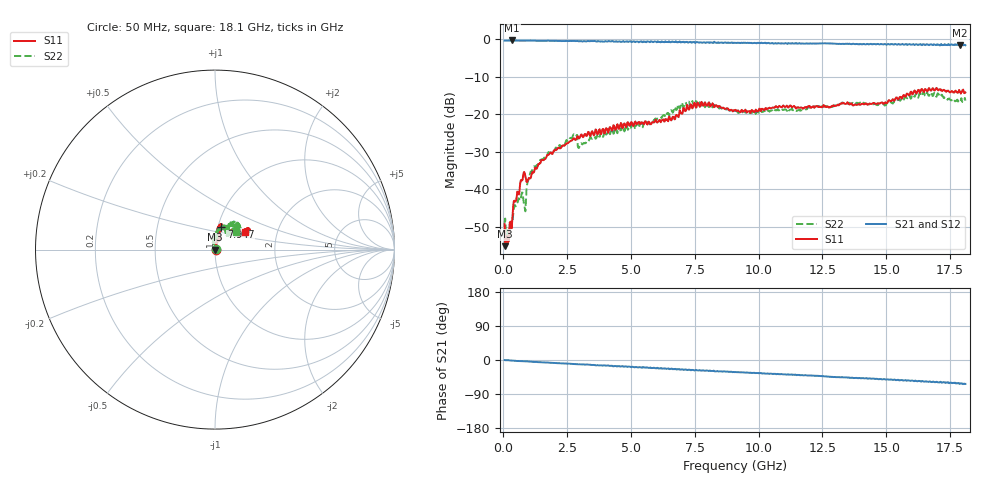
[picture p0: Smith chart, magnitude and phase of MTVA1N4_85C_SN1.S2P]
! Network Analyzer HP8720D.06.14 Serial No. US36140669
! 12 Jan 2005  09:00:05
! Frequency  S11  S21  S12  S22
# HZ  S  DB R 50
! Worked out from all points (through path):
!   801 points, 50 MHz to 18.1 GHz, reference 50 ohm
!   highest |S21| = -0.36 dB at 343.3 MHz (marker M1); lowest = -1.7 dB at 17.9 GHz (marker M2)
!   group delay of S21, straight-line fit = 9.33 ps
!   lowest |S11| = -55.1 dB at 72.56 MHz (marker M3), VSWR 1.00, Z = 50.1 - j0.101 ohm
!   |S11| at or under -10 dB: start of sweep to end of sweep
!   |S22| runs from -53.5 to -14.1 dB; largest |S21 - S12| = 0.032
!   S11 on the Smith chart (normalised r, x): 50 MHz: 1.01, -0.00; 7.947 GHz: 1.04, +0.27; 18.1 GHz: 1.37, +0.28
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5e7  -49.23 -2.3  -0.41 -0.2  -0.39 -0.6  -48.90 34.6
7.25625e7  -55.10 -34.8  -0.43 -0.4  -0.40 -0.7  -47.76 -15.5
1.628125e8  -52.34 58.2  -0.41 -0.5  -0.41 -0.9  -50.81 43.9
3.433125e8  -48.82 71.7  -0.36 -1.5  -0.38 -1.8  -48.94 57.1
5.238125e8  -41.96 87.7  -0.42 -2.6  -0.41 -2.8  -43.70 71.9
7.494375e8  -37.50 80.7  -0.46 -3.2  -0.44 -3.4  -40.84 69.7
8.6225e8  -36.39 60.8  -0.44 -3.5  -0.42 -3.8  -45.83 115.4
1.020188e9  -37.08 70.6  -0.43 -4.0  -0.41 -4.4  -36.63 109.2
1.22325e9  -34.88 84.5  -0.44 -5.2  -0.44 -5.4  -34.00 103.8
1.787312e9  -30.69 79.7  -0.45 -7.1  -0.44 -7.2  -30.08 100.8
2.689812e9  -26.97 74.7  -0.51 -10.3  -0.49 -10.7  -26.26 102.7
3.073375e9  -25.41 74.2  -0.56 -11.7  -0.52 -11.9  -27.88 98.6
4.043562e9  -23.77 68.3  -0.63 -14.9  -0.55 -14.6  -25.35 97.5
6.074188e9  -21.97 75.8  -0.68 -22.5  -0.67 -22.3  -21.21 85.4
7.066938e9  -18.28 76.4  -0.76 -26.1  -0.72 -25.5  -18.12 71.5
7.946875e9  -17.70 74.0  -0.96 -27.6  -0.84 -28.4  -17.40 55.7
9.075e9  -18.86 79.3  -1.00 -31.6  -0.92 -32.0  -19.14 48.0
1.209838e10  -18.09 66.6  -1.18 -41.1  -1.14 -41.5  -18.06 60.2
1.509919e10  -16.28 35.5  -1.36 -51.9  -1.23 -51.5  -17.14 62.5
1.652062e10  -13.28 31.4  -1.58 -57.1  -1.35 -56.8  -15.09 46.5
1.789694e10  -14.03 27.7  -1.70 -61.7  -1.71 -62.2  -16.68 46.3
1.81e10  -14.21 30.0  -1.64 -63.1  -1.63 -64.3  -16.38 41.1
